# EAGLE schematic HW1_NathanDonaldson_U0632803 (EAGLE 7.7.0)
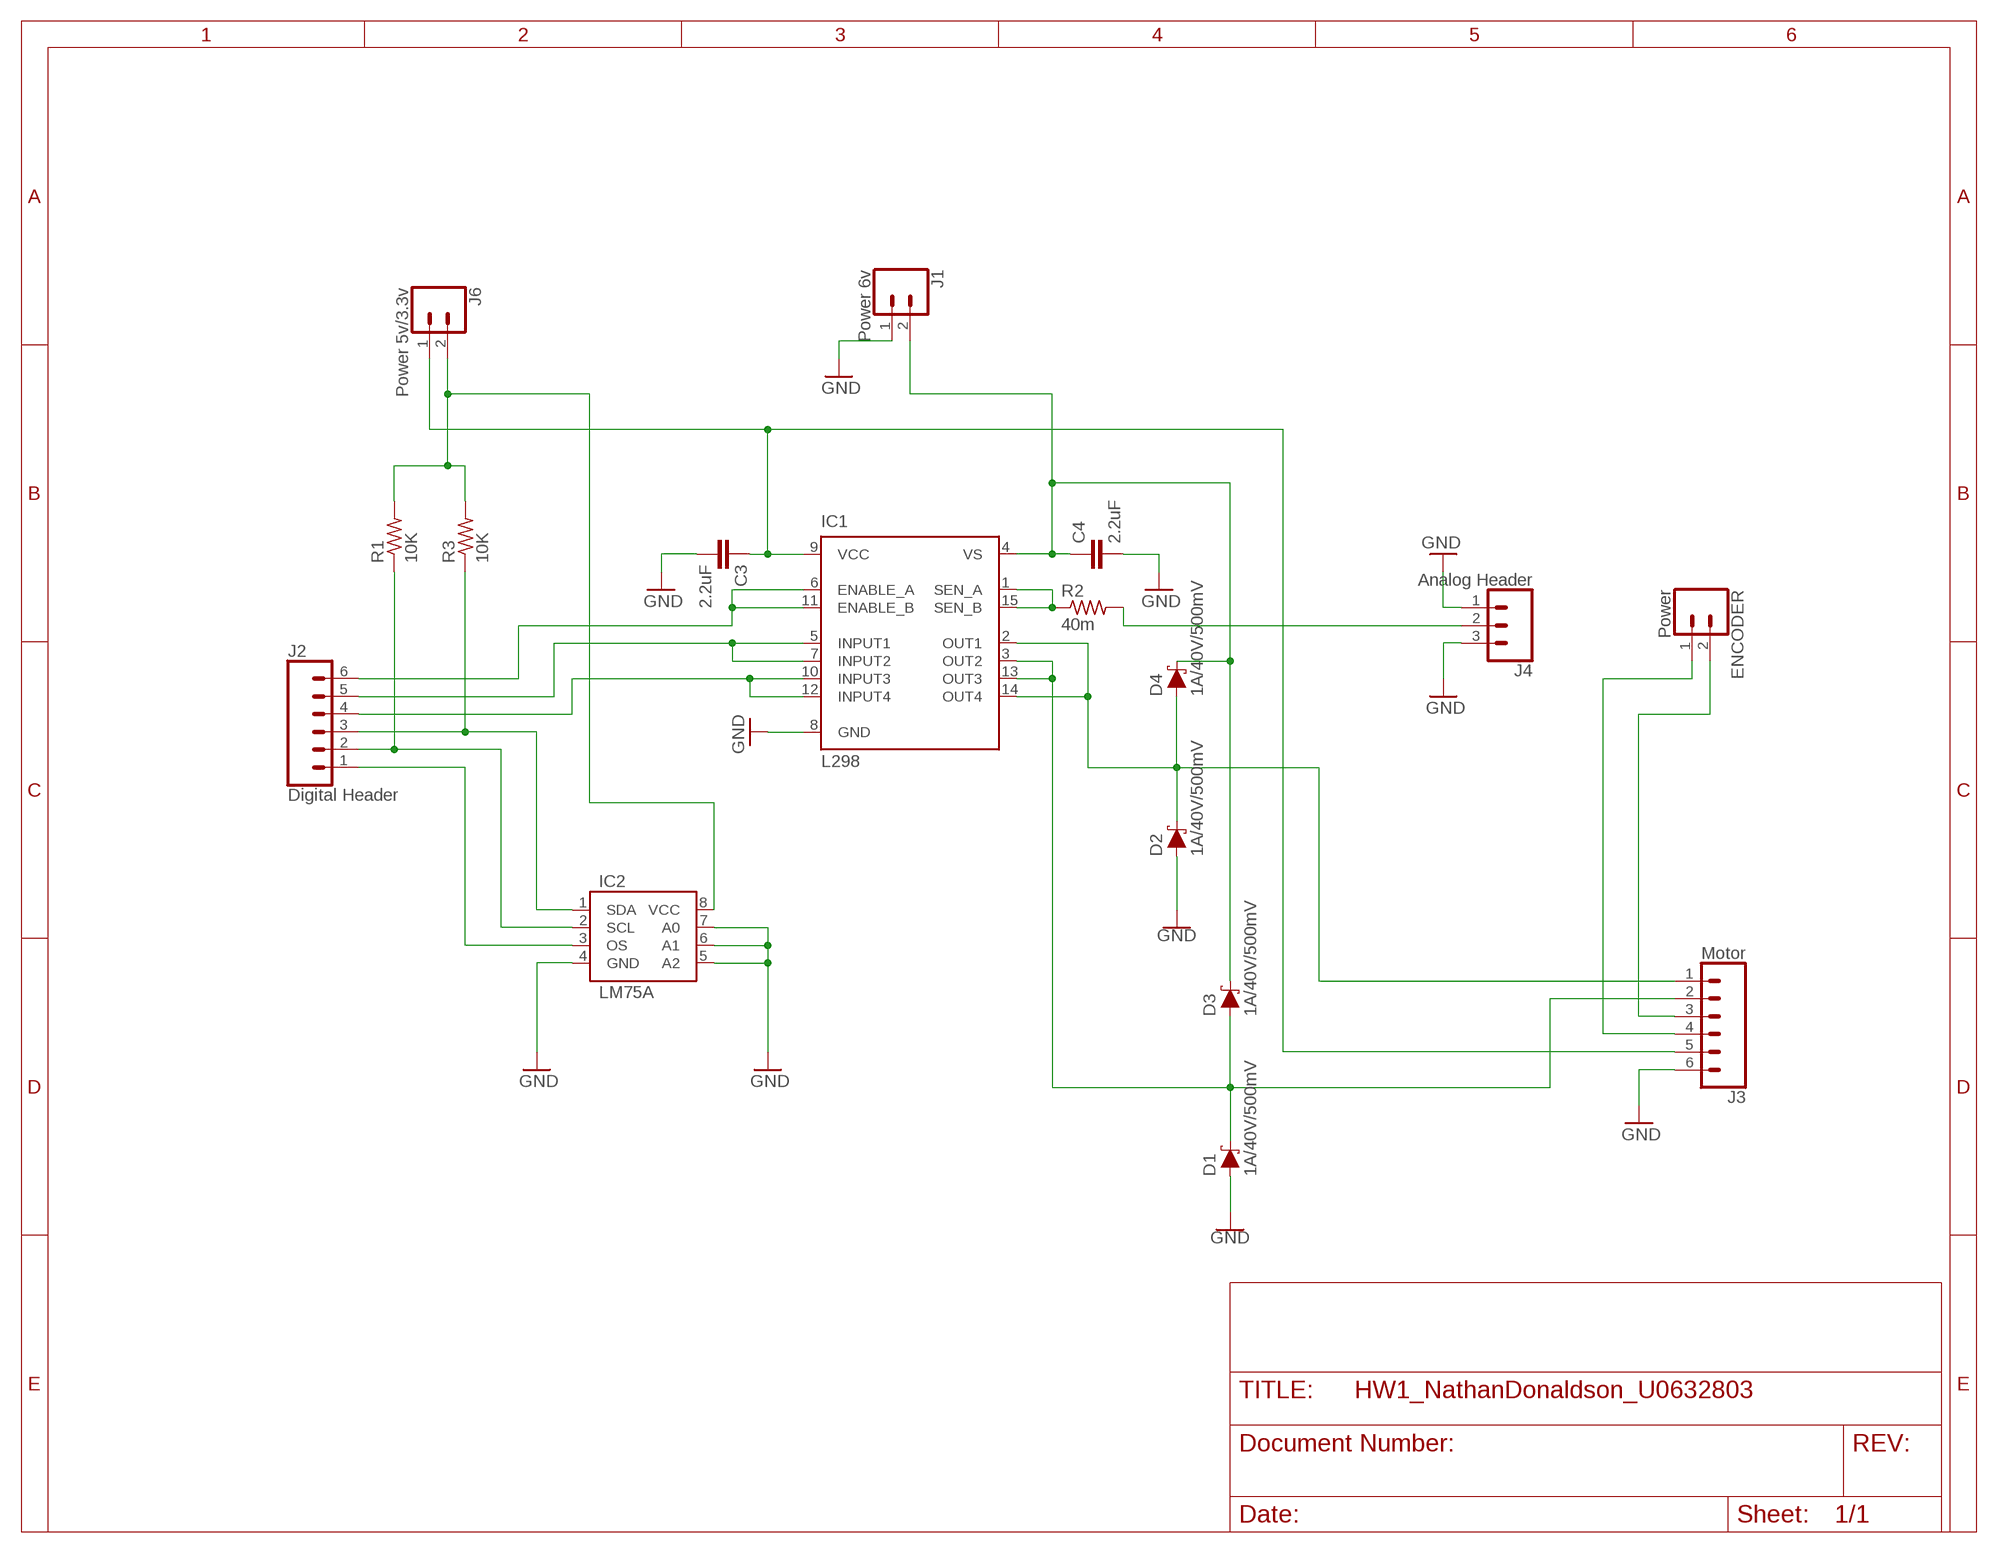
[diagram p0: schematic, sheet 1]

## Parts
C3  2.2uF  2.2UF-CERCAP-10009  [1206]
C4  2.2uF  2.2UF-CERCAP-10009  [1206]
D1  1A/40V/500mV  DIODE-SCHOTTKY-SS14  [SMA-DIODE]
D2  1A/40V/500mV  DIODE-SCHOTTKY-SS14  [SMA-DIODE]
D3  1A/40V/500mV  DIODE-SCHOTTKY-SS14  [SMA-DIODE]
D4  1A/40V/500mV  DIODE-SCHOTTKY-SS14  [SMA-DIODE]
ENCODER  Power  CONN_02  [1X02]
IC1  L298  [MULTIWATT-15]
IC2  LM75A  [SO8]
J1  Power 6v  CONN_02  [1X02]
J2  Digital Header  CONN_06LOCK  [1X06_LOCK]
J3  Motor  CONN_06LOCK  [1X06_LOCK]
J4  Analog Header  CONN_03  [1X03]
J6  Power 5v/3.3v  CONN_02  [1X02]
R1  10K  R-US_R1206  [R1206]
R2  40m  R-US_R1206  [R1206]
R3  10K  R-US_R1206  [R1206]

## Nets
GND: C3.2 C4.2 D1.A D2.A IC1.8(GND) IC2.4(GND) IC2.5(A2) IC2.6(A1) IC2.7(A0) J1.1 J3.6 J4.1 J4.3
N$1: J4.2 R2.2
N$2: ENCODER.2 J3.3
N$3: IC1.6(ENABLE_A) IC1.11(ENABLE_B) J2.6
N$4: ENCODER.1 J3.4
N$6: IC1.5(INPUT1) IC1.7(INPUT2) J2.5
N$7: IC1.10(INPUT3) IC1.12(INPUT4) J2.4
N$8: IC2.1(SDA) J2.3 R3.1
N$9: IC2.2(SCL) J2.2 R1.1
N$10: IC2.3(OS) J2.1
N$11: IC2.8(VCC) J6.2 R1.2 R3.2
N$12: IC1.1(SEN_A) IC1.15(SEN_B) R2.1
N$13: C3.1 IC1.9(VCC) J3.5 J6.1
N$16: D2.C D4.A IC1.2(OUT1) IC1.14(OUT4) J3.1
N$17: D1.C D3.A IC1.3(OUT2) IC1.13(OUT3) J3.2
N$19: C4.1 D3.C D4.C IC1.4(VS) J1.2

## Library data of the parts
C3 C4 = SparkFun-Retired:2.2UF-CER: 2.2uF Ceramic SMT; PROD_ID: CAP-10009
D1-D4 = SparkFun-DiscreteSemi:DIODE-SCHOTTKY: Schottky diode; PROD_ID: DIO-08053
ENCODER J1 J6 = SparkFun-Connectors:CONN_02: Multi connection point. Often used as Generic Header-pin footprint for 0.1 inch spaced/style header connections
IC1 = st-microelectronics:L298: DUAL FULL-BRIDGE DRIVER; MPN: L298N; OC_FARNELL: 1589425; OC_NEWARK: 32M1527
IC2 = nxp:LM75A
J2 J3 = SparkFun-Connectors:CONN_06: Multi connection point. Often used as Generic Header-pin footprint for 0.1 inch spaced/style header connections On any of the 0.1 inch spaced packages, you can populate with these: Break Away Headers - Straight (PRT-00116) Break Away Male Headers - Right Angle (PRT-00553) Female Headers (PRT-00115)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
J4 = SparkFun-Connectors:CONN_03: Multi connection point. Often used as Generic Header-pin footprint for 0.1 inch spaced/style header connections On any of the 0.1 inch spaced packages, you can populate with these: Break Away Headers - Straight (PRT-00116) Break Away Male Headers - Right Angle (PRT-00553) Female Headers (PRT-00115)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
R1-R3 = rcl:R-US_: RESISTOR, American symbol

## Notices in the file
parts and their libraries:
SparkFun-Retired: Licensing: Creative Commons ShareAlike 4.0 International - https://creativecommons.org/licenses/by-sa/4.0
